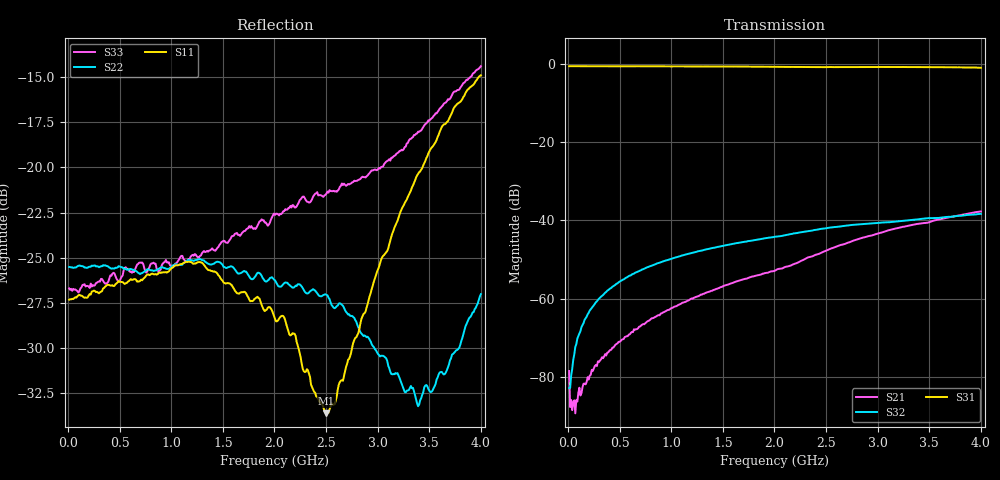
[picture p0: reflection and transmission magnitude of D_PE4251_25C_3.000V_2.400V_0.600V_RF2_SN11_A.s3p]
! Device ID: PE4251_SoldCshunt_081809
! Dir: c:\Test Bench Repositories\Bench_Software_CVI_Version_8\trunk\PSC 4Port_VNA Bench\datalog\4250\TEST\PE4251_SoldCshunt_081809\25C\3p000000\RF2
! Serial: 11
! Insertion: A
! Temp: 25C
! VDD: 3.000
! Control_Hi: 80.000
! Control_Lo: 20.000
! Logic State: RF2
! Port 1: RFC
! Port 2: RF1
! Port 3: RF2
! V1 = 0.60
! V2 = 0.60
! V3 = 0.60
! IDD: 4.326110e-05
! FILE NAME
! DATE 08/18/09  20:12
! CORRECTED  DATA
#  Hz  S  RI  R  50.00
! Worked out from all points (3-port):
!   401 points, 10 MHz to 4 GHz, reference 50 ohm
!   strongest paths, dB at 10 MHz, 1.008 GHz, 2.005 GHz, 3.002 GHz, 4 GHz:
!     S31: -0.6, -0.6, -0.7, -0.7, -0.9
!     S32: -82.9, -49.8, -44.2, -40.7, -38.3
!     S21: -78.5, -62.4, -52.9, -43.4, -37.7
!   lowest |S11| = -33.6 dB at 2.504 GHz (marker M1), VSWR 1.04, Z = 50.5 - j2.03 ohm
!   |S11| at or under -10 dB: start of sweep to end of sweep
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1e7  0.043 -0.000774  0.00011 -3.84e-06  0.9375 -0.003
     -7.73e-06 -0.000118  0.053 -0.00091  -4.32e-06 -3.09e-05
     0.9373 -0.00435  -1.44e-05 6.99e-05  0.0462 0.000272
8.98e7  0.0439 0.0011  1.73e-05 -5.63e-05  0.9384 -0.0323
        2.09e-05 -4.32e-05  0.0532 -0.00125  3.69e-05 0.000296
        0.939 -0.0323  3.82e-05 0.000305  0.0454 -0.000949
1.79575e8  0.0435 0.00192  2.55e-06 -8.25e-05  0.9362 -0.063
           4.22e-07 -8.53e-05  0.0527 -0.00155  6.21e-05 0.000581
           0.9362 -0.0635  5.82e-05 0.000582  0.0469 0.000293
2.99275e8  0.0446 0.00325  -3.76e-05 -0.000146  0.9317 -0.1052
           -4.39e-05 -0.000148  0.0528 -0.00257  8.93e-05 0.000985
           0.9315 -0.1043  8.55e-05 0.000992  0.0483 -0.000765
4.888e8  0.0484 0.00172  -0.000162 -0.000213  0.9203 -0.1682
         -0.000164 -0.000225  0.053 -0.00457  0.00015 0.0016
         0.9205 -0.1676  0.000153 0.0016  0.0483 -0.00413
1.0474e9  0.0524 -0.0108  -0.00074 -0.000317  0.8665 -0.3486
          -0.000734 -0.000311  0.0527 -0.0114  0.000505 0.00334
          0.867 -0.3484  0.000496 0.00333  0.0532 -0.0103
2.005e9  0.0353 -0.0142  -0.00224 -0.000388  0.6958 -0.6049
         -0.00224 -0.000387  0.0481 -0.00714  0.00117 0.00605
         0.6966 -0.6053  0.00116 0.00608  0.0665 -0.0322
2.50375e9  0.00558 -0.02  -0.00403 -0.000814  0.5843 -0.7029
           -0.00402 -0.000831  0.0444 -0.000219  0.00158 0.00779
           0.5866 -0.703  0.0016 0.00777  0.0529 -0.0661
3.391525e9  -0.0879 -0.0387  -0.00899 0.00106  0.3452 -0.846
            -0.00898 0.00107  0.0127 0.0177  0.00237 0.01
            0.3472 -0.846  0.00235 0.01  -0.0279 -0.1225
4e9  -0.1783 -0.0269  -0.0125 0.00371  0.1302 -0.8875
     -0.0125 0.0037  -0.0264 0.0359  0.00251 0.0118
     0.1312 -0.8868  0.0025 0.0119  -0.135 -0.1351
